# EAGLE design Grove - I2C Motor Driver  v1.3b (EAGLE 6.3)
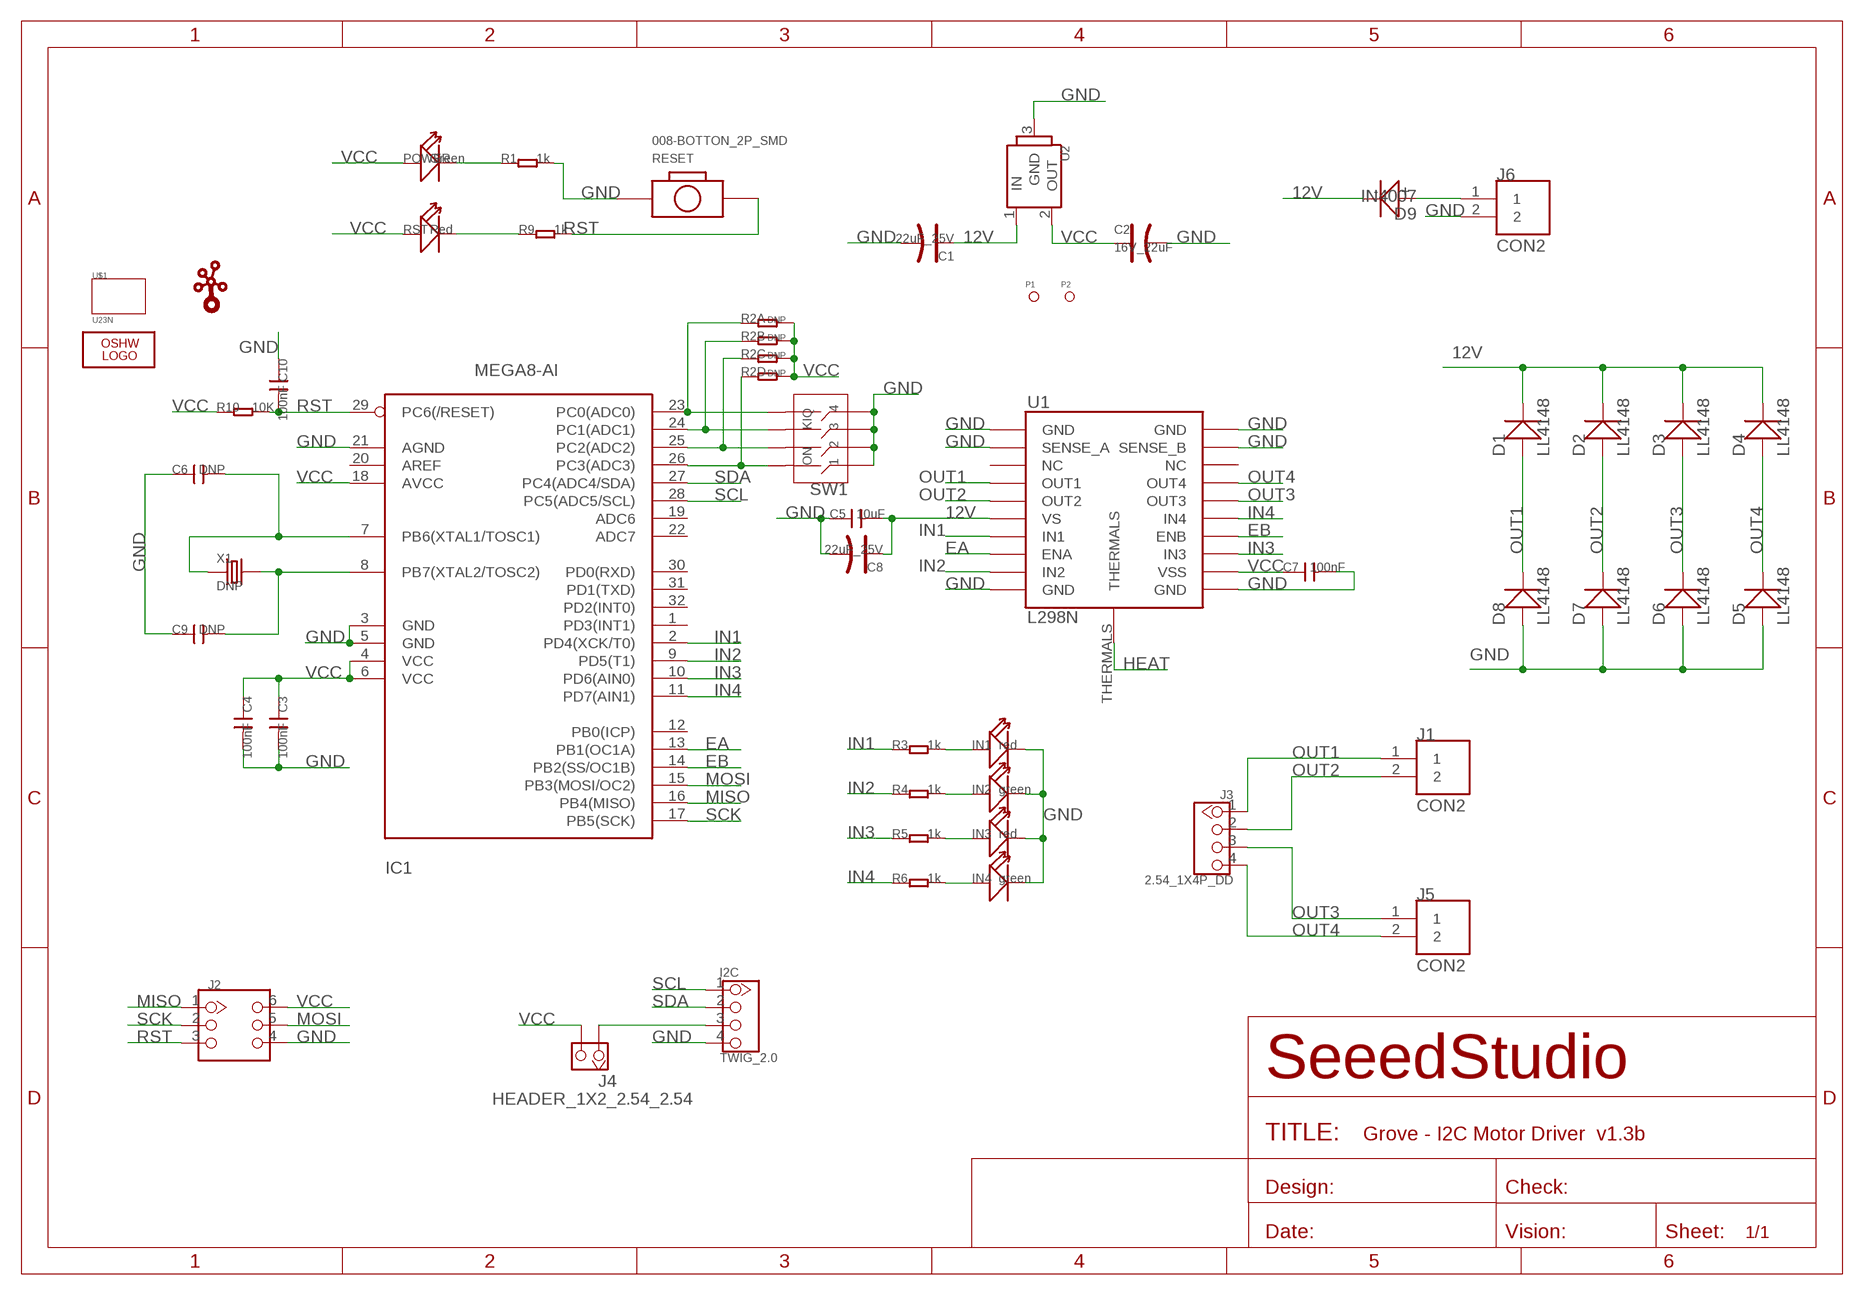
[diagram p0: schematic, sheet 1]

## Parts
C1  22uF_25V  CAP-AVX-C  [AVX-C]
C2  16V_22uF  CAP-AVX-B  [AVX-B]
C3  100nF  C-0603  [0603]
C4  100nF  C-0603  [0603]
C5  10uF  C-0805  [0805]
C6  DNP  006-C30*35  [0603_S]
C7  100nF  C-0603  [0603]
C8  22uF_25V  CAP-AVX-C  [AVX-C]
C9  DNP  006-C30*35  [0603_S]
C10  100nF  006-C30*35  [0603_S]
D1  LL4148  D'1206'  [SOD123]
D2  LL4148  D'1206'  [SOD123]
D3  LL4148  D'1206'  [SOD123]
D4  LL4148  D'1206'  [SOD123]
D5  LL4148  D'1206'  [SOD123]
D6  LL4148  D'1206'  [SOD123]
D7  LL4148  D'1206'  [SOD123]
D8  LL4148  D'1206'  [SOD123]
D9  IN4007  010-D2010  [D2010@1]
I2C  TWIG_2.0  [2.0_1X4]
IC1  MEGA8-AI  [TQFP32-08]
IN1  red  007-LED0603  [D0603]
IN2  green  007-LED0603  [D0603]
IN3  red  007-LED0603  [D0603]
IN4  green  007-LED0603  [D0603]
J1  CON2  [CON2]
J2  HEADER-2X3P-60/35MIL  [2X3P-2.54-65/35MIL]
J3  2.54_1X4P_DD  [CK_1X4]
J4  HEADER_1X2_2.54_2.54  [65*35]
J5  CON2  [CON2]
J6  CON2  [CON2]
LOGO2  LOGO-OSHW-FILLX0200-NT  [OSHW_FILLX200_NOTEXT]
P1  PAD-MARK  [ROUND-MARK-1.0]
P2  PAD-MARK  [ROUND-MARK-1.0]
POWER  Green  007-LED0603  [D0603]
R1  1k  005-R0603  [0603-1]
R2  DNP  R-4R-1206  [1206-8-3.3X2.4]
R3  1k  005-R0603  [0603-1]
R4  1k  005-R0603  [0603-1]
R5  1k  005-R0603  [0603-1]
R6  1k  005-R0603  [0603-1]
R9  1k  005-R0603  [0603-1]
R10  10K  005-R0603  [0603-1]
RESET  008-BOTTON_2P_SMD  [BOTTON_1]
RST  Red  007-LED0603  [D0603]
SW1  SWITCH-KM-04'KM-04'  [8P-SMD-11.8X6.8X3.3H]
U1  L298N  L298_BRIDGE_DRIVER  [POWERSO20]
U2  78M05-TO252  [TO252]
U$1  U23N  [U2*3N]
U$3  TWIGLOGOTWIGLOGO_SMALL  [TWIGLOGO_SMALL]
X1  DNP  CRYSTAL-5032  [2P-SMD-5X3.2]

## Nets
12V: C1.+ C5.2 C8.+ D1.- D2.- D3.- D4.- D9.- U1.P$6(VS) U2.1(IN)
EA: IC1.13(PB1(OC1A)) U1.P$8(ENA)
EB: IC1.14(PB2(SS/OC1B)) U1.P$14(ENB)
GND: C1.- C2.- C3.2 C4.2 C5.1 C6.1 C7.2 C8.- C9.1 C10.1 D5.+ D6.+ D7.+ D8.+ I2C.4 IC1.3(GND) IC1.5(GND) IC1.21(AGND) IN1.- IN2.- IN3.- IN4.- J2.4 J6.2 R1.2 RESET.1 SW1.1 SW1.2 SW1.3 SW1.4 U1.P$1(GND) U1.P$2(SENSE_A) U1.P$10(GND) U1.P$11(GND) U1.P$19(SENSE_B) U1.P$20(GND) U2.3(GND)
HEAT: U1.THERMALS
IN1: IC1.2(PD4(XCK/T0)) R3.1 U1.P$7(IN1)
IN2: IC1.9(PD5(T1)) R4.1 U1.P$9(IN2)
IN3: IC1.10(PD6(AIN0)) R5.1 U1.P$13(IN3)
IN4: IC1.11(PD7(AIN1)) R6.1 U1.P$15(IN4)
MISO: IC1.16(PB4(MISO)) J2.1
MOSI: IC1.15(PB3(MOSI/OC2)) J2.5
N$1: IN3.+ R5.2
N$2: I2C.3 J4.1
N$3: POWER.- R1.1
N$4: IC1.23(PC0(ADC0)) R2.1 SW1.5
N$5: IC1.24(PC1(ADC1)) R2.2 SW1.6
N$7: IC1.25(PC2(ADC2)) R2.3 SW1.7
N$8: C6.2 IC1.7(PB6(XTAL1/TOSC1)) X1.1
N$9: C9.2 IC1.8(PB7(XTAL2/TOSC2)) X1.2
N$10: R9.1 RST.-
N$11: IC1.26(PC3(ADC3)) R2.4 SW1.8
N$12: D9.+ J6.1
N$14: IN1.+ R3.2
N$15: IN2.+ R4.2
N$17: IN4.+ R6.2
OUT1: D1.+ D8.- J1.1 J3.1 U1.P$4(OUT1)
OUT2: D2.+ D7.- J1.2 J3.2 U1.P$5(OUT2)
OUT3: D3.+ D6.- J3.3 J5.1 U1.P$16(OUT3)
OUT4: D4.+ D5.- J3.4 J5.2 U1.P$17(OUT4)
RST: C10.2 IC1.29(PC6(/RESET)) J2.3 R9.2 R10.2 RESET.P$2
SCK: IC1.17(PB5(SCK)) J2.2
SCL: I2C.1 IC1.28(PC5(ADC5/SCL))
SDA: I2C.2 IC1.27(PC4(ADC4/SDA))
VCC: C2.+ C3.1 C4.1 C7.1 IC1.4(VCC) IC1.6(VCC) IC1.18(AVCC) J2.6 J4.2 POWER.+ R2.5 R2.6 R2.7 R2.8 R10.1 RST.+ U1.P$12(VSS) U2.2(OUT)
Unconnected: IC1.1(PD3(INT1)) IC1.12(PB0(ICP)) IC1.19(ADC6) IC1.20(AREF) IC1.22(ADC7) IC1.30(PD0(RXD)) IC1.31(PD1(TXD)) IC1.32(PD2(INT0)) U1.P$3(NC) U1.P$18(NC)

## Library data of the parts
C1 C2 C8 = Discrete:CAP*: Electrolytic Capacitors,Tantalum Capacitors and Super Capacitors
C3-C5 C7 = Discrete:C*: Ceramic Capacitors
C6 C9 C10 = Discrete:006-C*: Ceramic Capacitors
D1-D8 = Discrete:D*
D9 = Discrete:010-D*
I2C = CONNECTER:TWIG_2.0
IC1 = IC:MEGA8: MICROCONTROLLER 8 Kbytes FLASH 1 kbytes SRAM 512 bytes EEPROM USART 6-channel 10 bit ADC 2-channel 8 bit ADC
IN1-IN4 POWER RST = Discrete:007-LED*
J1 J5 J6 = 2pin:CON2
J2 = Connector:HEADER-2X3P
J3 = Connector:2.54_1X4P
J4 = Connector:HEADER_1X2_2.54
LOGO2 = Logo:LOGO-OSHW-FILL
P1 P2 = Discrete:PAD-MARK; PARTNO: DNP
R1 R3-R6 R9 R10 = Discrete:005-R*
R2 = Discrete:R-4R*: Resistor Array
RESET = Discrete:008-BOTTON_2P
SW1 = Discrete:SWITCH-KM-04
U1 = ICs:L298_BRIDGE_DRIVER
U2 = IC:78M05: 0.5A Three Terminal Positive Voltage Regulators http://pdf1.alldatasheet.com/datasheet-pdf/view/31368/TOSHIBA/78M05/+21_79UPLRhpDDdCDytD+/datasheet.pdf
U$1 = twig_template1:U2*3N
U$3 = seeedleo:TWIGLOGO
X1 = Discrete:CRYSTAL*: CRYSTAL

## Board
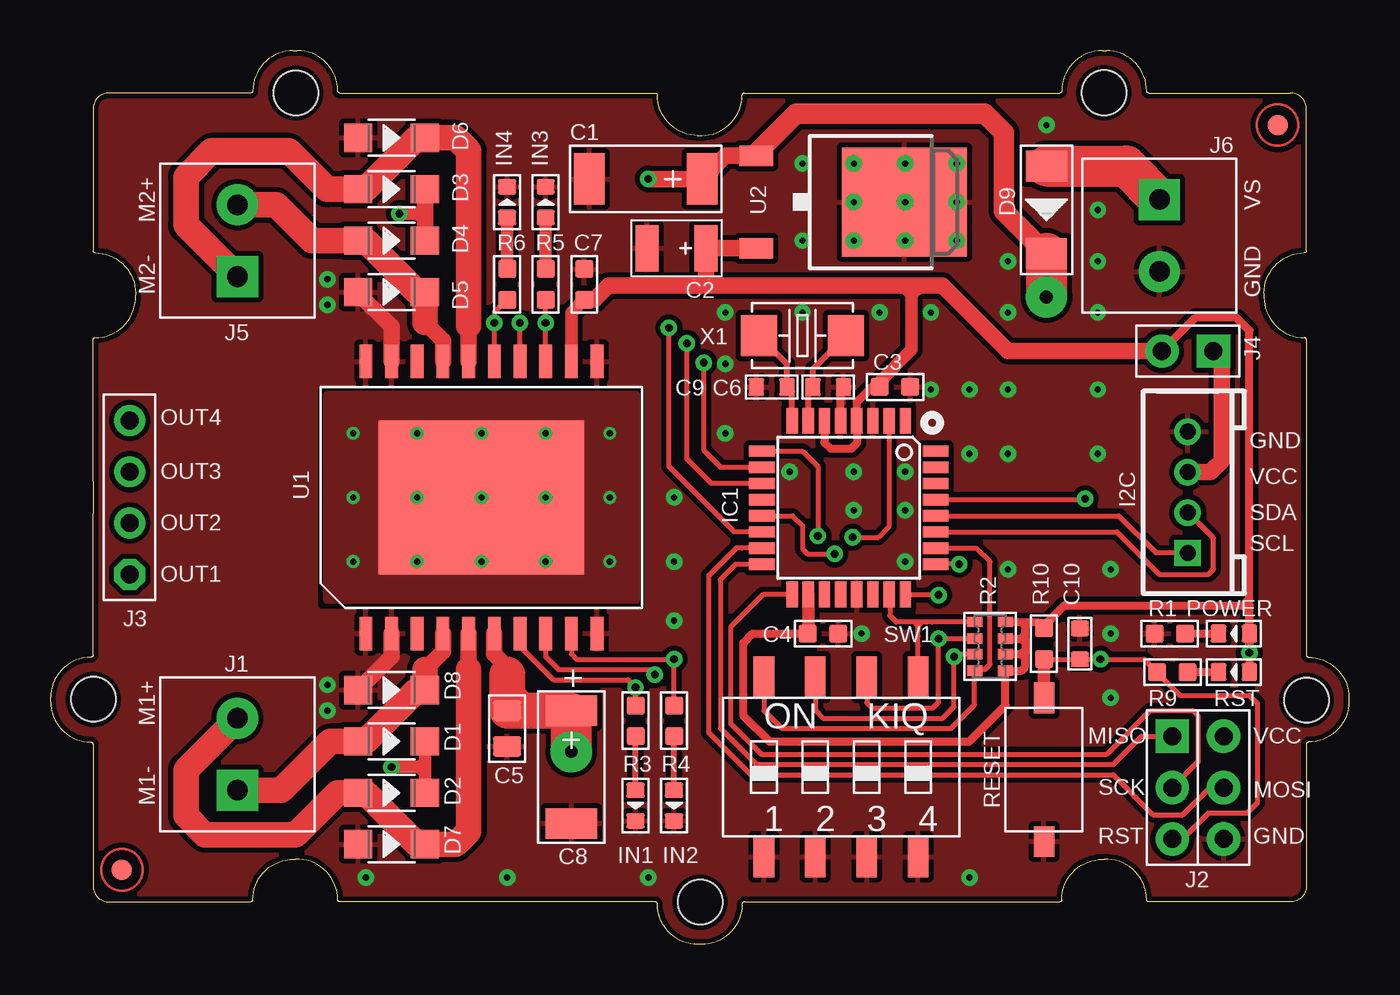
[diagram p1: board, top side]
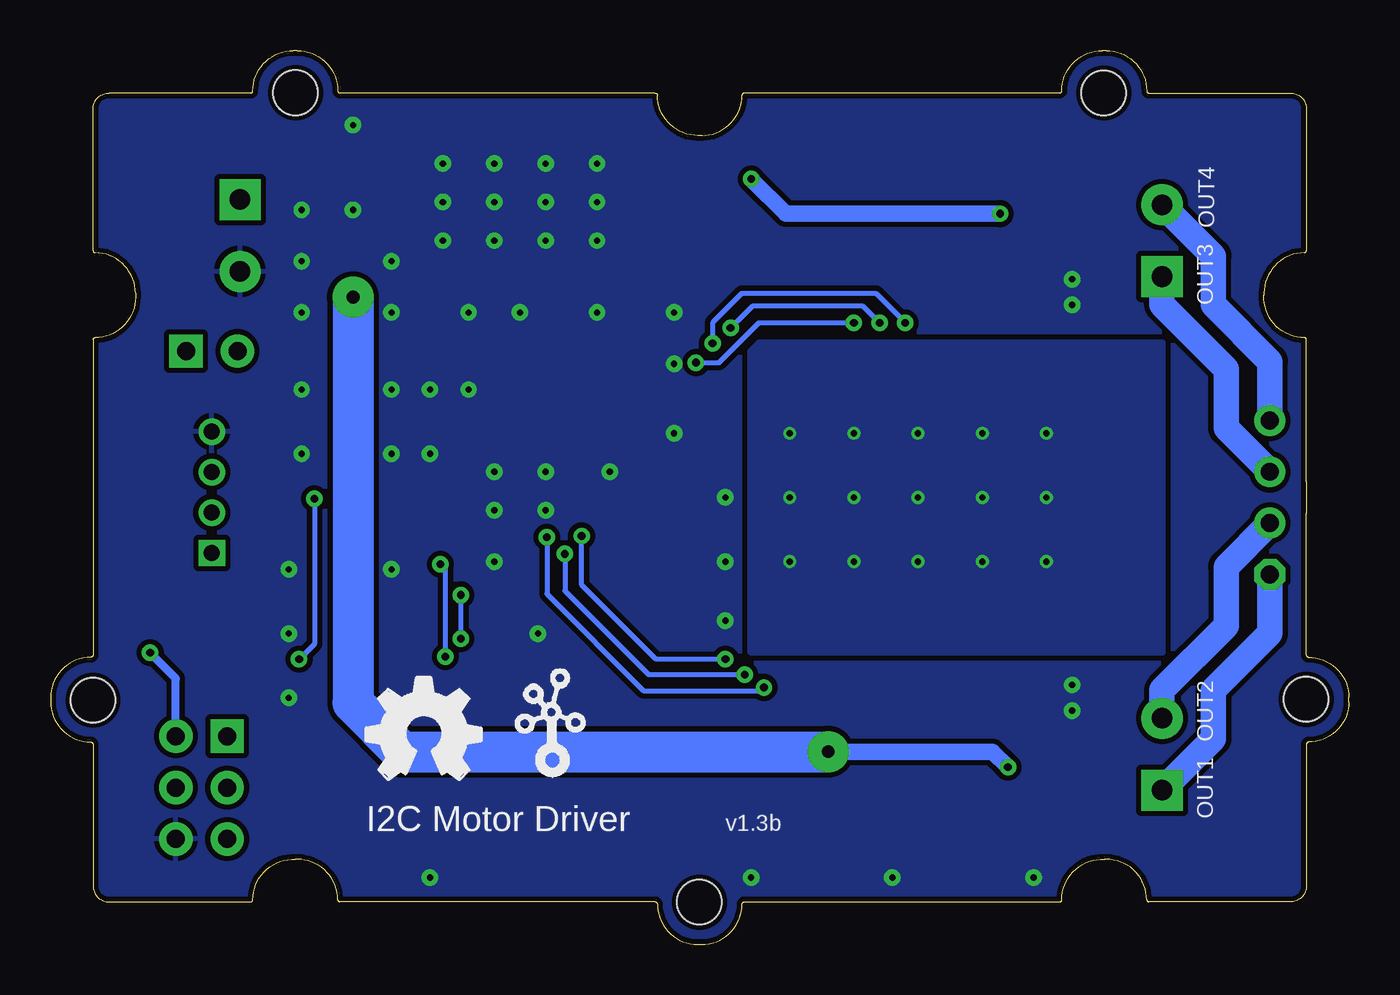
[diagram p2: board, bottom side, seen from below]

Size 64.2 x 44.2 mm. Coordinates in mm from the lower left corner, seen from the top.
Copper layers (1*16): Top 0.035mm / dielectric 1.5mm / Bottom 0.035mm
Design rules "default": minimum track width 6mil, minimum drill 12mil, track to track 6mil, track to pad 6mil, pad to pad 6mil, via to via 6mil, smd to smd 0mil, copper to edge 10mil, drill to drill 10mil, minimum pad ring 10mil, minimum via ring 6mil, stop-mask expansion 2mil, vias tented up to drill 25mil, thermal gap 10mil
tRestrict: area 16.1,28.5 to 16.3,29.2; area 16.1,15 to 16.3,15.7

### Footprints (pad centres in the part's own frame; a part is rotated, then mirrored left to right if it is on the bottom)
AVX-C = smd 1.524 x 2.54: + -2.794,0; - 2.794,0
AVX-B = smd 1.143 x 2.286: + -1.46,0; - 1.46,0
0603 = smd 0.889 x 0.889: 1 -0.762,0; 2 0.762,0
0805 = smd 1.016 x 1.397: 1 -0.889,0; 2 0.889,0
0603_S = smd 0.762 x 0.889: 1 -0.762,0; 2 0.762,0
SOD123 = smd 1.397 x 1.397: + -1.651,0; - 1.651,0
D2010@1 = smd 1.524 x 2.032: + -2.159,0; - 2.159,0
2.0_1X4 = drill 0.8 pad 1.27 square: 1 -3,0 | drill 0.8 pad 1.27: 2 -1,0; 3 1,0; 4 3,0
TQFP32-08 = smd 1.27 x 0.559: 1 -4.293,2.8; 2 -4.293,2; 3 -4.293,1.2; 4 -4.293,0.4; 5 -4.293,-0.4; 6 -4.293,-1.2; 7 -4.293,-2; 8 -4.293,-2.8; 17 4.293,-2.8; 18 4.293,-2; 19 4.293,-1.2; 20 4.293,-0.4; 21 4.293,0.4; 22 4.293,1.2; 23 4.293,2; 24 4.293,2.8 | smd 0.559 x 1.27: 9 -2.8,-4.293; 10 -2,-4.293; 11 -1.2,-4.293; 12 -0.4,-4.293; 13 0.4,-4.293; 14 1.2,-4.293; 15 2,-4.293; 16 2.8,-4.293; 25 2.8,4.293; 26 2,4.293; 27 1.2,4.293; 28 0.4,4.293; 29 -0.4,4.293; 30 -1.2,4.293; 31 -2,4.293; 32 -2.8,4.293
D0603 = smd 0.762 x 0.889: + -0.762,0; - 0.762,0
CON2 = drill 1.016 pad 2.032 square: 1 0,1.778 | drill 1.016 pad 2.032: 2 0,-1.778
2X3P-2.54-65/35MIL = drill 0.889 pad 1.651 square: 1 -1.27,2.54 | drill 0.889 pad 1.651: 2 -1.27,0; 3 -1.27,-2.54; 4 1.27,-2.54; 5 1.27,0; 6 1.27,2.54
CK_1X4 = drill 0.889 pad 1.524 octagon: 1 0,3.81 | drill 0.889 pad 1.524: 2 0,1.27; 3 0,-1.27; 4 0,-3.81
65*35 = drill 0.889 pad 1.651 square: 1 0,1.27 | drill 0.889 pad 1.651: 2 0,-1.27
ROUND-MARK-1.0 = smd 1.016 x 1.016: P$1 0,0
0603-1 = smd 0.889 x 0.889: 1 -0.762,0; 2 0.762,0
1206-8-3.3X2.4 = smd 0.508 x 0.762: 1 -1.206,-0.762; 2 -0.381,-0.762; 3 0.381,-0.762; 4 1.206,-0.762; 5 1.206,0.762; 6 0.381,0.762; 7 -0.381,0.762; 8 -1.206,0.762
BOTTON_1 = smd 1.524 x 1.016: 1 -3.556,0; P$2 3.556,0
8P-SMD-11.8X6.8X3.3H = smd 1.016 x 2.032: 1 -3.81,-4.445; 2 -1.27,-4.445; 3 1.27,-4.445; 4 3.81,-4.445; 5 3.81,4.445; 6 1.27,4.445; 7 -1.27,4.445; 8 -3.81,4.445
POWERSO20 = smd 1.651 x 0.635: P$1 -6.731,5.715; P$2 -6.731,4.445; P$3 -6.731,3.175; P$4 -6.731,1.905; P$5 -6.731,0.635; P$6 -6.731,-0.635; P$7 -6.731,-1.905; P$8 -6.731,-3.175; P$9 -6.731,-4.445; P$10 -6.731,-5.715; P$11 6.731,-5.715; P$12 6.731,-4.445; P$13 6.731,-3.175; P$14 6.731,-1.905; P$15 6.731,-0.635; P$16 6.731,0.635; P$17 6.731,1.905; P$18 6.731,3.175; P$19 6.731,4.445; P$20 6.731,5.715 | smd 7.62 x 10.16: THERMALS 0,0
TO252 = smd 1.016 x 1.651: 1 -2.286,-4.826; 2 2.286,-4.826 | smd 5.4 x 6.2: 3 0,2.5
U2*3N = hole 2.2: -0.017,20.015; -30.005,10.02; 29.985,9.983; 19.98,-20.005; -19.983,-20.015
2P-SMD-5X3.2 = smd 1.778 x 2.032: 1 -2.159,0; 2 2.159,0

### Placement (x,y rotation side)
C1  29.43,37.85 180 top
C2  30.96,34.42 180 top
C3  41.75,27.56 0 top
C4  38.2,15.37 0 top
C5  22.58,10.67 90 top
C6  38.45,27.56 180 top
C7  26.39,32.64 90 top
C8  25.75,8.77 270 top
C9  35.66,27.56 0 top
C10  50.9,14.86 270 top
D1  16.86,10.04 0 top
D2  16.86,7.5 0 top
D3  16.86,37.34 0 top
D4  16.86,34.8 0 top
D5  16.86,32.26 0 top
D6  16.86,39.88 0 top
D7  16.86,4.96 0 top
D8  16.86,12.58 0 top
D9  49.25,36.32 270 top
I2C  56.23,22.35 90 top
IC1  39.47,21.59 270 top
IN1  28.93,6.86 270 top
IN2  30.83,6.86 270 top
IN3  24.48,36.7 90 top
IN4  22.58,36.7 90 top
J1  9.24,9.4 180 top
J2  56.74,7.75 0 top
J3  3.91,22.1 180 top
J4  56.23,29.34 270 top
J5  9.24,34.8 180 top
J6  54.83,35.05 0 top
LOGO2  48.58,8.14 0 bottom
P1  3.53,3.69 0 top
P2  60.67,40.52 0 top
POWER  58.52,15.37 180 top
R1  55.34,15.37 180 top
R2  46.45,14.73 270 top
R3  28.93,11.05 270 top
R4  30.83,11.05 270 top
R5  24.48,32.64 90 top
R6  22.58,32.64 90 top
R9  55.47,13.46 180 top
R10  49.12,14.86 270 top
RESET  49.12,8.64 90 top
RST  58.52,13.46 180 top
SW1  39.09,8.77 0 top
U1  21.3,22.1 90 top
U2  39.72,36.7 270 top
U$1  32.1,22.1 180 top
U$3  41.62,8.13 0 bottom
X1  37.18,30.1 180 top

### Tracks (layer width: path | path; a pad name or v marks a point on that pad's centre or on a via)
12V  (via drill 0.38 pad 0.81, 0.64 pad 2.03)
  Top 0.61: v17.24,36.13 18.13,36.13 | 18.13,36.13 18.51,36.13 18.51,36.52 18.45,36.58 18.45,36.45 18.13,36.13 | 18.13,36.13 18.45,35.82 | D1.- 18.51,9.02 | 18.51,9.02 18.51,8.77 | 18.51,8.77 18.51,8.45 | 18.51,8.45 D2.- | v16.86,8.77 18.19,8.77 | 18.26,8.77 18.51,8.77 | 18.19,8.77 18.26,8.77 | 18.26,8.77 18.51,9.02 | 18.19,8.77 18.51,8.45
  Top 0.813: U1.P$6 21.94,14.35 22.58,13.72 22.58,13.34 | D3.- 18.51,36.13 D4.- | v29.56,37.85 C1.+ 33.37,38.99 U2.1
  Top 1.016: D9.- 47.15,36.26 47.15,40.13 46.2,41.09 36.86,41.09 34.89,39.12 U2.1
  Top 1.778: 23.27,11.56 C5.2 22.58,13.34 | 23.27,11.56 C8.+ 25.75,11.31 | 23.27,11.56 22.64,12.19
  Top 2.032: D9.- v49.25,32.01 | v25.75,9.53 25.75,11.31
  Bottom 0.813: v17.24,36.13 27.85,36.13 v29.56,37.85 | v25.75,9.53 17.62,9.53 v16.86,8.77
  Bottom 2.032: v25.75,9.53 46.83,9.53 49.25,11.94 v49.25,32.01
EA  (via drill 0.38 pad 0.81)
  Top 0.254: U1.P$8 24.48,14.23 25.12,13.59 29.56,13.59 | 29.56,13.59 29.81,13.34 | IC1.13 36.69,21.19 37.18,20.7 37.18,19.56 37.43,19.31 v38.77,19.31 | 29.56,13.59 29.62,13.59 v29.88,13.34
  Bottom 0.254: v38.77,19.31 38.77,17.48 34.62,13.34 v29.88,13.34
EB  (via drill 0.38 pad 0.81)
  Top 0.254: IC1.14 33.81,20.39 30.58,23.63 v30.58,30.48 | U1.P$14 v23.21,30.74
  Bottom 0.254: v30.58,30.48 29.5,31.56 24.04,31.56 v23.21,30.74
GND  (via drill 0.3 pad 0.81)
  Top 0.406: IC1.5 39.07,27.42 C6.1
  Top 0.813: U1.P$19 16.86,30.55 15.15,32.26 | U1.P$2 16.86,14.23 D8.+
  other vias: 39.72,38.61 42.26,38.61 44.8,38.61 39.72,36.7 42.26,36.7 44.8,36.7 44.8,34.8 42.26,34.8 39.72,34.8 49.25,40.52 49.25,36.32 51.78,36.32 51.78,33.78 51.78,31.24 47.34,31.24 47.34,33.78 43.53,31.24 43.53,27.43 47.34,27.43 45.44,27.43 45.44,24.26 47.34,24.26 51.78,24.26 51.78,27.43 40.99,31.24 33.37,31.24 33.37,28.7 33.37,25.28 39.72,21.46 39.72,23.37 42.26,23.37 42.26,21.46 42.26,18.93 47.34,18.54 52.42,18.54 52.42,15.37 52.42,12.19 37.18,38.61 37.18,36.7 37.18,34.8 40.1,15.37 36.55,23.37 37.18,31.24 15.59,3.3 13.69,12.83 22.58,3.3 29.56,3.3 45.44,3.3 13.69,11.56 30.83,16 30.83,18.93 30.83,22.1 13.69,31.62 13.69,32.9
  pour Bottom: -5.49,44.58 -4.22,44.58 -4.22,43.31 -5.49,43.31
  pour Top (isolate 0.254, rank 6): -0.28,44.33 64.48,44.33 64.48,-0.12 -0.28,-0.12
  pour Bottom (isolate 0.254, rank 6): -0.28,44.33 64.48,44.33 64.48,-0.12 -0.28,-0.12
HEAT  (via drill 0.3 pad 0.64)
  other vias: 21.3,22.1 18.13,22.1 14.96,22.1 24.48,22.1 27.66,22.1 27.66,25.28 24.48,25.28 21.3,25.28 18.13,25.28 14.96,25.28 14.96,18.93 18.13,18.93 21.3,18.93 24.48,18.93 27.66,18.93
  pour Top (isolate 0.406, no thermals): 13.69,27.18 28.93,27.18 28.93,17.02 13.69,17.02
  pour Bottom (isolate 0.406, no thermals): 9.24,29.72 29.56,29.72 29.56,14.48 9.24,14.48
IN1  (via drill 0.38 pad 0.81)
  Top 0.254: U1.P$7 23.21,14.73 24.86,13.08 28.54,13.08 v28.93,12.7 R3.1 | IC1.2 41.47,20.67 40.93,20.13 v39.66,20.13
  Bottom 0.254: v39.66,20.13 39.66,17.33 34.87,12.54 29.09,12.54 v28.93,12.7
IN2  (via drill 0.38 pad 0.81)
  Top 0.254: U1.P$9 25.75,14.35 26,14.1 v30.83,14.1 R4.1 | IC1.9 37.17,24.39 37.94,23.62 v37.94,20.2
  Bottom 0.254: v30.83,14.1 34.26,14.1 37.94,17.78 v37.94,20.2
IN3  (via drill 0.38 pad 0.81)
  Top 0.254: IC1.10 33.15,23.59 32.29,24.45 v32.29,28.77 | U1.P$13 v24.48,30.74 R5.1
  Bottom 0.254: v32.29,28.77 31.15,28.77 29.18,30.74 v24.48,30.74
IN4  (via drill 0.38 pad 0.81)
  Top 0.254: IC1.11 32.68,22.79 31.46,24.01 v31.46,29.72 | U1.P$15 v21.94,30.74 21.94,31.24 R6.1
  Bottom 0.254: v31.46,29.72 31.46,30.74 30.01,32.2 23.4,32.2 v21.94,30.74
MISO
  Top 0.254: IC1.16 33.87,18.79 33.12,18.04 33.12,10.67 34.89,8.89 52.55,8.89 53.94,10.29 J2.1
MOSI
  Top 0.254: 34.16,19.59 IC1.15 33.91,19.59 32.55,18.23 32.55,10.48 34.64,8.38 52.55,8.38 54.52,6.42 55.98,6.42 57.31,7.75 J2.5
N$1
  Top 0.61: R5.2 IN3.+
N$2
  Top 0.813: J4.1 57.91,28.93 57.91,23.9 57.36,23.35 I2C.3
N$3
  Top 0.406: R1.1 POWER.-
N$4
  Top 0.254: SW1.5 42.9,14.73 | 42.9,14.73 42.9,15.24 | R2.1 43.59,15.94 43.31,15.94 | 42.9,14.73 42.9,15.5 | 42.9,15.5 42.9,15.62 | IC1.23 41.5,17.27 41.5,17.02 41.5,16.26 41.82,15.94 43.31,15.94 | 42.9,15.5 42.9,15.75 | 42.9,15.75 43.02,15.88 43.09,15.94 43.31,15.94 | 42.9,15.5 42.9,15.75 | 42.9,15.75 42.77,15.88
N$5  (via drill 0.38 pad 0.81)
  Top 0.254: SW1.6 40.36,11.94 40.61,11.69 43.63,11.69 43.91,11.97 v43.91,15.12 R2.2 | v43.91,17.27 42.29,17.27 IC1.24
  Bottom 0.254: v43.91,15.12 v43.91,17.27
N$7  (via drill 0.38 pad 0.81)
  Top 0.254: SW1.7 37.81,11.56 38.2,11.18 44.11,11.18 44.67,11.75 v44.67,14.23 44.8,14.35 R2.3 | v44.93,18.8 43.78,18.8 43.78,18.79 IC1.25
  Bottom 0.254: v44.67,14.23 44.67,18.54 v44.93,18.8
N$8
  Top 0.305: IC1.7 37.47,27.34 C6.2 37.69,28.45 X1.1
N$9
  Top 0.305: IC1.8 36.67,27.31 C9.2 36.42,28.7 X1.2
N$10
  Top 0.406: R9.1 RST.-
N$11
  Top 0.254: SW1.8 35.27,11.57 36.17,10.67 44.52,10.67 45.69,11.84 R2.4 | R2.4 45.69,13.59 | R2.4 45.69,13.59 | 45.69,13.59 46.2,13.59 46.45,13.85 46.45,18.93 45.82,19.56 45.78,19.59 IC1.26
N$12
  Top 2.032: D9.+ 53.18,38.48 J6.1
N$14
  Top 0.305: IN1.+ 28.93,10.04 R3.2
N$15
  Top 0.305: IN2.+ R4.2
N$17
  Top 0.61: R6.2 IN4.+
OUT1
  Top 0.813: U1.P$4 19.4,14.48 18.51,13.59
  Top 1.27: 18.51,13.59 D8.- 18.13,12.58 15.59,10.04 D1.+ 13.81,10.04 11.4,7.62 J1.1
  Bottom 1.27: J1.1 6.7,10.16 6.7,12.58 3.91,15.37 J3.1
OUT2
  Top 0.813: U1.P$5 20.67,13.59
  Top 1.27: 20.67,13.59 20.67,5.59 20.04,4.96 D7.- 18.13,4.96 15.59,7.5 D2.+ 14.19,7.5 12.12,5.42 7.63,5.42 6.7,6.35 6.7,8.64 J1.2
  Bottom 1.27: J3.2 6.07,18.67 6.07,15.75 9.24,12.58 J1.2
OUT3
  Top 0.813: U1.P$16 20.67,30.61
  Top 1.27: 20.67,30.61 20.67,39.25 20.04,39.88 D6.- 18.13,39.88 15.59,37.34 D3.+ 13.69,37.34 11.78,39.25 7.97,39.25 6.7,37.98 6.7,35.56 J5.1
  Bottom 1.27: J3.3 6.07,25.53 6.07,28.45 9.24,31.62 J5.1
OUT4
  Top 0.813: U1.P$17 19.4,29.85 18.51,30.74
  Top 1.27: 18.51,30.74 D5.- 18.13,32.26 15.59,34.8 D4.+ 12.92,34.8 11.15,36.58 J5.2
  Bottom 1.27: J5.2 6.7,34.04 6.7,31.62 3.91,28.83 J3.4
RST  (via drill 0.38 pad 0.81)
  Top 0.254: J2.3 55.98,5.21 57.25,6.48 59.15,6.48 59.66,6.99 59.66,11.94 59.28,12.32 55.84,12.32 R9.2 54.07,14.1 v51.91,14.1 | R10.2 C10.2 | C10.2 v51.91,14.1 | IC1.29 51.11,21.99 v51.15,22.04 | v51.91,14.1 C10.2
  Top 0.61: RESET.P$2 R10.2
  Bottom 0.254: v51.15,22.04 51.15,14.86 v51.91,14.1
SCK
  Top 0.254: IC1.17 35.24,17.3 33.62,15.69 33.62,10.92 35.15,9.4 52.23,9.4 54.39,11.56 56.48,11.56 56.74,11.31 56.74,9.02 J2.2
SCL
  Top 0.254: IC1.28 52.82,21.19 54.64,19.37 54.66,19.35 I2C.1
SDA
  Top 0.254: IC1.27 52.73,20.39 54.82,18.3 57.26,18.3 57.5,18.54 57.5,20.09 I2C.2
VCC  (via drill 0.38 pad 0.81)
  Top 0.254: 47.91,15.12 47.98,15.18
  Top 0.305: 48.19,15.94 48.19,15.58 48.17,15.56 48.17,15.69 47.91,15.94 | 48.23,15.43 47.98,15.18 | 47.91,15.12 48.17,14.86 | 48.17,14.61 47.91,14.35 48.17,14.1
  Top 0.406: POWER.+ RST.+ | R2.8 47.91,15.94 48.19,15.94 | 48.19,15.94 48.42,15.94 | 48.42,15.94 48.8,15.94 R10.1 49.12,15.75 50.13,16.77 58.96,16.77 | 48.19,15.94 48.19,15.71 | 48.19,15.12 48.19,14.35 | R2.5 47.99,13.53 48.19,13.73 48.19,14.35 | R2.6 47.91,14.35 48.19,14.35 | R2.7 47.91,15.12 48.19,15.12 | 59.28,16.26 POWER.+ | C4.1 34.72,15.37 34.26,14.91 34.26,11.31 35.54,10.03 45.43,10.03 47.21,11.81 R2.5 | 47.21,13.59 R2.5 | C3.1 40.61,27.56 39.87,26.82 IC1.4 39.87,24.79 39.59,24.51 38.58,24.51 38.27,24.82 IC1.6 | POWER.+ 59.28,16.51 | 59.28,16.51 59.28,16.77 | 59.28,16.77 59.28,30.36 58.64,30.99 56.61,30.99 J4.2 | v59.28,14.42 POWER.+ | 59.02,16.77 59.28,16.77 | 58.96,16.77 59.21,17.02 | 58.96,16.77 59.02,16.77 | 59.02,16.77 59.28,16.51 | 48.19,15.12 48.19,15.71 | 48.19,15.71 48.42,15.94
  Top 0.61: IC1.18 37.47,15.4 C4.1 | C3.1 40.99,27.82 42.58,29.4 42.58,32.26 42.26,32.58 | 42.13,32.58 42.58,32.13 42.96,32.51 | 32.42,32.64 32.55,32.64 32.61,32.7 | U1.P$12 25.75,31.24 C7.1
  Top 0.813: 32.48,32.58 27.85,32.58 27.59,32.58 26.89,31.88 C7.1 | 32.48,32.58 42.13,32.58 42.26,32.58 44.1,32.58 47.34,29.34 J4.2 | 32.48,32.58 32.42,32.64 C2.+ U2.2 | 32.16,32.64 32.42,32.9 32.61,32.7
  Bottom 0.406: J2.6 58.01,13.15 v59.28,14.42

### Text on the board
tPlace: VS | M2+ | GND | M2- | OUT4 | GND | OUT3 | VCC | SDA | OUT2 | SCL | OUT1 | + | M1+ | MISO | VCC | M1- | SCK | MOSI | RST | GND
bPlace: OUT4 | OUT3 | OUT2 | OUT1 | v1.3b | I2C Motor Driver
